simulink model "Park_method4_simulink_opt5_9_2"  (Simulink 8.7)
settings: Solver=ode45  StartTime=0.0  StopTime=0.5  FixedStep=5e-7  RelTol=1e-3
libraries: powerlib x1

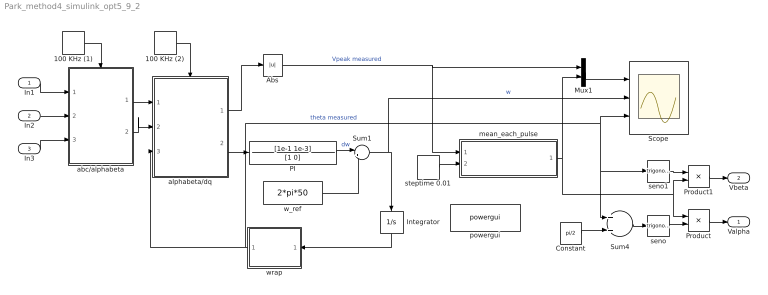
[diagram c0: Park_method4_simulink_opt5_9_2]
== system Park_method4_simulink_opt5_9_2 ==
  In1 : Inport
  In2 : Inport  Port=2
  In3 : Inport  Port=3
  100 KHz (1) : DiscretePulseGenerator  PulseType=Time based  Period=10e-6  PulseWidth=50
  100 KHz (2) : DiscretePulseGenerator  PulseType=Time based  Period=10e-6  PulseWidth=50
  Abs : Abs
  Constant : Constant  Value=pi/2
  Integrator : Integrator
  Mux1 : Mux  Inputs=2
  PI : TransferFcn  Numerator=[1e-1 1e-3]  Denominator=[1 0]
  Product : Product
  Product1 : Product
  Scope : Scope  NumInputPorts=3
  Sum1 : Sum  Inputs=|++
  Sum4 : Sum
  abc/alphabeta : Subsystem
  alphabeta/dq : Subsystem
  mean_each_pulse : MATLAB Function  TreatAsAtomicUnit=on
  powergui : powerlib/powergui  Priority=1  SimulationMode=Discrete  SolverType=Tustin  SampleTime=5e-7  frequency=60  SPID=off  DisableSnubberDevices=off  DisableRonSwitches=off  DisableVfSwitches=off  SwTol=0  DisplayEquations=off  Interpol=off  ExternalGateDelay=off  methode=off  Ts=10  FunctionMessages=off  echomessages=off  HookPort=off  EnableUseOfTLC=off  x0status=blocks  frequencyindice=0  Pbase=100e6  ErrMax=1e-4  Iterations=50  UnitsV=kV  UnitsW=MW  buscounter=0  RestoreLinks=warning  ResistiveCurrentMeasurement=off  Frange=[0:2:500]  Ylog=off  Xlog=on  ShowGrid=off  save=off  variable=ZData  structure=0  ZoomFFT=off  StartTime=0.0  cycles=1  DisplayStyle=1  fundamental=60  FreqAxis=off  MaxFrequency=1000  frequencyindicesteady=1  RmsSteady=1  display=off
  seno : Trigonometry
  seno1 : Trigonometry
  steptime 0.01 : DiscretePulseGenerator  PulseType=Time based  Period=0.01
  w_ref : Constant  Value=2*pi*50
  wrap : MATLAB Function  TreatAsAtomicUnit=on
  Valpha : Outport
  Vbeta : Outport  Port=2
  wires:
  Integrator/1 -> wrap/1(theta)
  PI/1 -> Sum1/1  "dw"
  wrap/1(theta2) -> alphabeta/dq/3(theta), Sum4/1, seno1/1, Scope/3  "theta measured"
  w_ref/1 -> Sum1/2
  Sum1/1 -> Integrator/1, Scope/2  "w"
  Abs/1 -> mean_each_pulse/1(u), Mux1/1  "Vpeak measured"
  seno/1 -> Product/2
  Product/1 -> Valpha/1
  Sum4/1 -> seno/1
  Constant/1 -> Sum4/2
  Product1/1 -> Vbeta/1
  seno1/1 -> Product1/1
  abc/alphabeta/1(alpha) -> alphabeta/dq/1(alpha)
  alphabeta/dq/1(Vd) -> Abs/1
  alphabeta/dq/2(Vq) -> PI/1
  100 KHz (2)/1 -> alphabeta/dq/Trigger
  abc/alphabeta/2(beta) -> alphabeta/dq/2(beta)
  100 KHz (1)/1 -> abc/alphabeta/Trigger
  In1/1 -> abc/alphabeta/1(a)
  In2/1 -> abc/alphabeta/2(b)
  In3/1 -> abc/alphabeta/3(c)
  steptime 0.01/1 -> mean_each_pulse/2(pulse)
  mean_each_pulse/1(mean_u) -> Product/1, Product1/2, Mux1/2
  Mux1/1 -> Scope/1

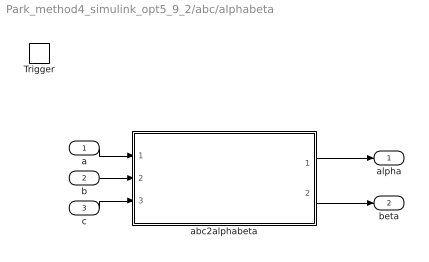
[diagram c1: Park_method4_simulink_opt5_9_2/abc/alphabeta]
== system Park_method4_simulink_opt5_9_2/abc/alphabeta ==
  a : Inport
  b : Inport  Port=2
  c : Inport  Port=3
  Trigger : TriggerPort  VariantControl=Variant
  abc2alphabeta : MATLAB Function  TreatAsAtomicUnit=on
  alpha : Outport
  beta : Outport  Port=2
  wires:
  abc2alphabeta/1(alpha) -> alpha/1
  c/1 -> abc2alphabeta/3(c)
  b/1 -> abc2alphabeta/2(b)
  a/1 -> abc2alphabeta/1(a)
  abc2alphabeta/2(beta) -> beta/1

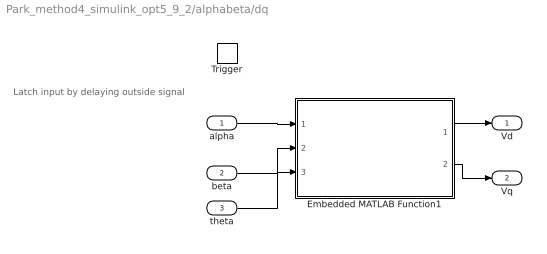
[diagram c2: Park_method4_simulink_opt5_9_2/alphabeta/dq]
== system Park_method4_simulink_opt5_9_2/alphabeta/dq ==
  note: Latch input by delaying outside signal
  alpha : Inport
  beta : Inport  Port=2
  theta : Inport  Port=3
  Trigger : TriggerPort  VariantControl=Variant
  Embedded MATLAB Function1 : MATLAB Function  TreatAsAtomicUnit=on
  Vd : Outport
  Vq : Outport  Port=2
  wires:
  alpha/1 -> Embedded MATLAB Function1/1(alpha)
  beta/1 -> Embedded MATLAB Function1/2(beta)
  theta/1 -> Embedded MATLAB Function1/3(theta)
  Embedded MATLAB Function1/1(Vd) -> Vd/1
  Embedded MATLAB Function1/2(Vq) -> Vq/1

== matlab function alphabeta//dq/Embedded
MATLAB Function1 ==
function [Vd,Vq]  = sinc(alpha, beta, theta)

% Variables persistentes (como 'static' en lenguaje C)
persistent oldTheta 
if isempty(oldTheta)
    oldTheta = 0;
   
    
end
% Transformacion


Vd=(alpha*cos(theta)+beta*sin(theta));
Vq=-alpha*sin(theta)+beta*cos(theta);
oldTheta = theta;

return
    
%end function

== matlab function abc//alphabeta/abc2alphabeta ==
function [alpha, beta] = abc_AlphaBetaGamma(a, b, c)

k1 = 2 / 3;
k2 = 1 / 3;
k3 = sqrt(3) / 3;

alpha = a * k1 - b * k2 - c * k2;
beta  =          b * k3 - c * k3;
% gamma = a * k2 + b * k2 + c * k2;
    
%end function

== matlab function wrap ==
function theta2   = wrap(theta)

% Variables persistentes (como 'static' en lenguaje C)

frame=floor(theta/(2*pi));
theta2=theta-frame*2*pi;



return
    
%end function

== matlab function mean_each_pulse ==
function mean_u   = mean_each_pulse(u , pulse)

persistent cont mean_last_iteration pulse_last mean_last_period;

if ( isempty(pulse_last) )
    pulse_last = 0;
end
if ( isempty(cont) )
    cont = 1;
end
if ( isempty(mean_last_iteration) )
    mean_last_iteration = 0;
end
if ( isempty(mean_last_period) )
    mean_last_period = 0;
end

% calculate only if pulse values 1

    
    % mean{n} = sum(xi)/n
    % = (x1 + x2 + ... + xn) / n
    % = (x1 + x2 + ... + x{n-1}) / (n - 1) * ((n - 1) / n) + xn / n
    % = mean{n-1} * ((n - 1) / n) + xn / n
    mean_last_iteration = mean_last_iteration  * ((cont - 1) / cont) + u / cont;
           
    cont = cont + 1;

if pulse == 1 && pulse_last == 0
    % restart cont
    cont = 1;
    mean_last_period = mean_last_iteration;
end

mean_u = mean_last_period;

pulse_last = pulse;
return

%end function
